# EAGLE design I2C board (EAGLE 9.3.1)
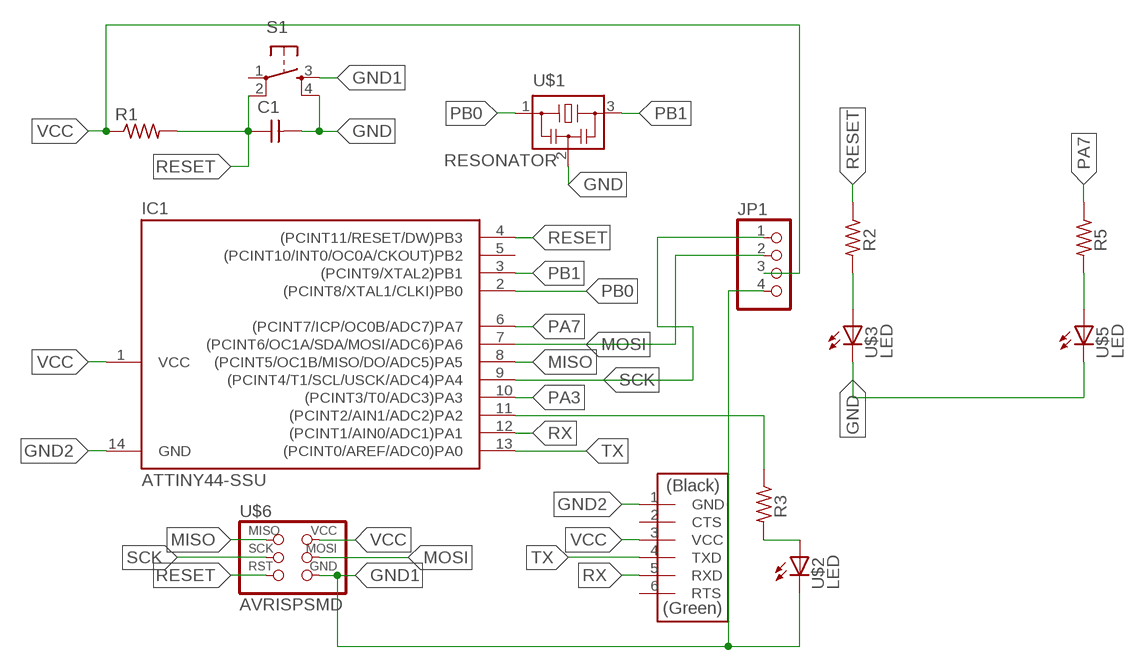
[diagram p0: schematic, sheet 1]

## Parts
C1  CAP-UNPOLARIZED  [C1206]
IC1  ATTINY44-SSU  [SOIC14]
JP1  PINHD-1X4  [1X04]
R1  RES-US1206  [R1206]
R2  RES-US1206  [R1206]
R3  RES-US1206  [R1206]
R5  RES-US1206  [R1206]
S1  6MM_SWITCH6MM_SWITCH  [6MM_SWITCH]
U$1  RESONATOR  [EFOBM]
U$2  LED  [LED1206]
U$3  LED  [LED1206]
U$5  LED  [LED1206]
U$6  AVRISPSMD  [2X03SMD]
U$7  FTDI-SMD-HEADER  [1X06SMD]

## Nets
GND: C1.2 S1.4(S1) U$1.2 U$3.2(C) U$5.2(C)
GND1: JP1.4 S1.3(S) U$2.2(C) U$6.6(GND)
GND2: IC1.14(GND) U$7.1(GND)
MISO: IC1.8((PCINT5/OC1B/MISO/DO/ADC5)PA5) U$6.1(MISO)
MOSI: IC1.7((PCINT6/OC1A/SDA/MOSI/ADC6)PA6) JP1.2 U$6.4(MOSI)
N$1: R3.2 U$2.1(A)
N$14: IC1.11((PCINT2/AIN1/ADC2)PA2) R3.1
N$20: R2.2 U$3.1(A)
N$23: R5.2 U$5.1(A)
PA3: IC1.10((PCINT3/T0/ADC3)PA3)
PA7: IC1.6((PCINT7/ICP/OC0B/ADC7)PA7) R5.1
PB0: IC1.2((PCINT8/XTAL1/CLKI)PB0) U$1.1
PB1: IC1.3((PCINT9/XTAL2)PB1) U$1.3
RESET: C1.1 IC1.4((PCINT11/RESET/DW)PB3) R1.2 R2.1 S1.2(P1) U$6.5(RST)
RX: IC1.12((PCINT1/AIN0/ADC1)PA1) U$7.5(RXD)
SCK: IC1.9((PCINT4/T1/SCL/USCK/ADC4)PA4) JP1.1 U$6.3(SCK)
TX: IC1.13((PCINT0/AREF/ADC0)PA0) U$7.4(TXD)
VCC: IC1.1(VCC) JP1.3 R1.1 U$6.2(VCC) U$7.3(VCC)
Unconnected: IC1.5((PCINT10/INT0/OC0A/CKOUT)PB2) S1.1(P) U$7.2(CTS) U$7.6(RTS)

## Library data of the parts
C1 = eagle_fab:CAP-UNPOLARIZED
IC1 = eagle_fab:ATTINY44
JP1 = pinhead:PINHD-1X4: PIN HEADER
R1-R3 R5 = eagle_fab:RES-US: Resistor (US Symbol)
S1 = eagle_fab:6MM_SWITCH: OMRON SWITCH
U$1 = eagle_fab:RESONATOR
U$2 U$3 U$5 = eagle_fab:LED: LED
U$6 = eagle_fab:AVRISP
U$7 = eagle_fab:FTDI-SMD-HEADER

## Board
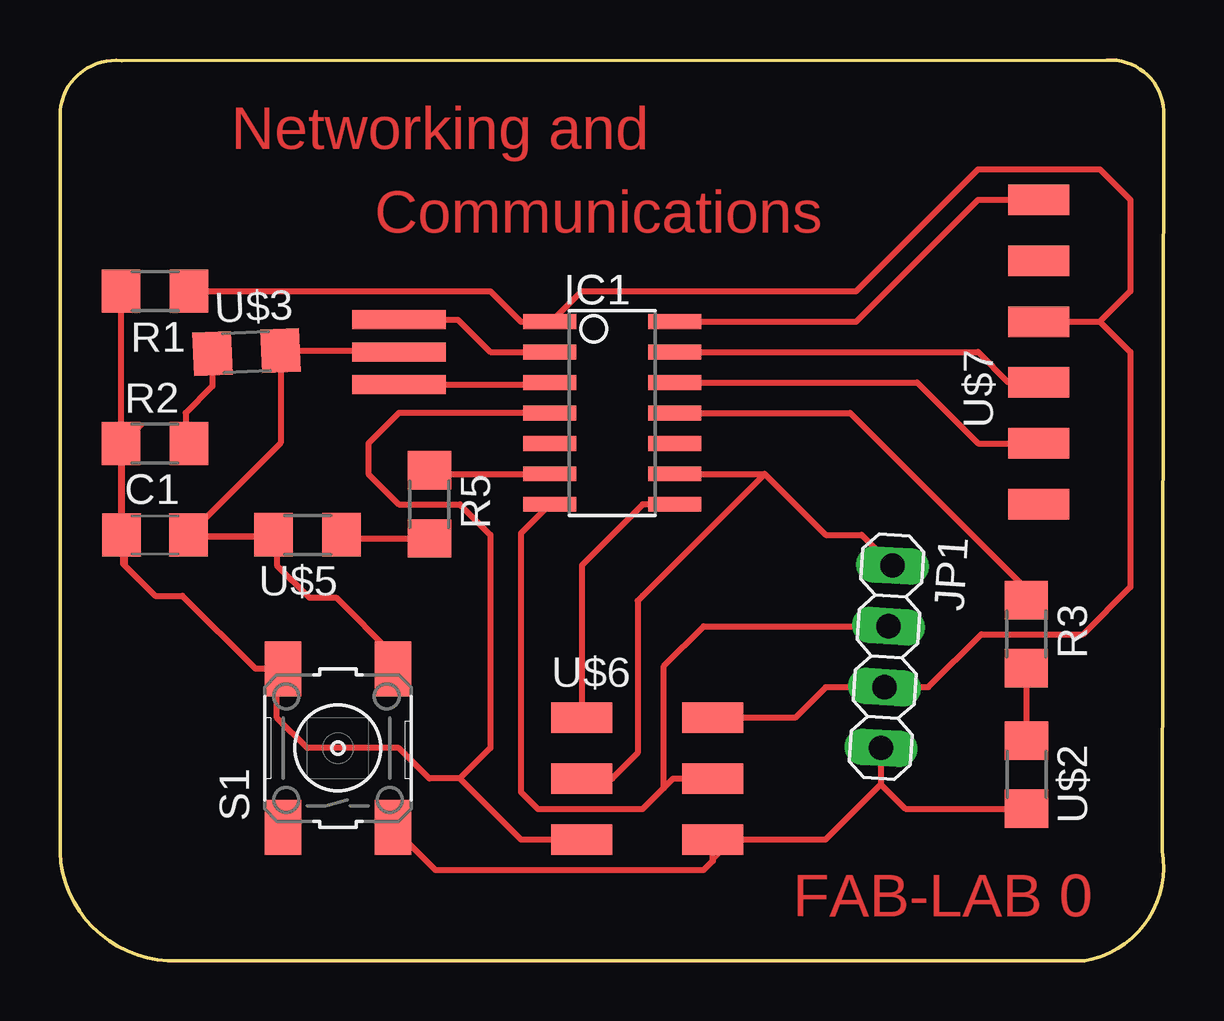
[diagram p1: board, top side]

Size 45.99 x 37.55 mm. Coordinates in mm from the lower left corner, seen from the top.
Outline: 0,35.44 arc-90 2.57,37.52 43.61,37.55 arc-90 45.99,35.44 45.93,4.59 arc-90 42.7,0 4.49,0.01 arc-90 0,4.96 0,35.44
Copper layers (1*16): Top 0.035mm / dielectric 1.5mm / Bottom 0.035mm
Design rules "default": minimum track width 6mil, minimum drill 0.35mm, track to track 6mil, track to pad 6mil, pad to pad 6mil, via to via 6mil, smd to smd 6mil, copper to edge 40mil, drill to drill 6mil, minimum pad ring 10mil, minimum via ring 8mil, stop-mask expansion 4mil, vias tented up to drill 0mil, thermal gap 10mil

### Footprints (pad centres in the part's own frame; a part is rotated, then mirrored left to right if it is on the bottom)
C1206 = smd 1.6 x 1.8: 1 -1.4,0; 2 1.4,0
SOIC14 = smd 0.61 x 2.21: 1 -3.81,-2.603; 2 -2.54,-2.603; 3 -1.27,-2.603; 4 0,-2.603; 5 1.27,-2.603; 6 2.54,-2.603; 7 3.81,-2.603; 8 3.81,2.603; 9 2.54,2.603; 10 1.27,2.603; 11 0,2.603; 12 -1.27,2.603; 13 -2.54,2.603; 14 -3.81,2.603
1X04 = drill 1.016 long: 1 -3.81,0; 2 -1.27,0; 3 1.27,0; 4 3.81,0
R1206 = smd 1.6 x 1.803: 1 -1.422,0; 2 1.422,0
6MM_SWITCH = smd 2.286 x 1.524: 1 -3.302,2.286; 2 3.302,2.286; 3 -3.302,-2.286; 4 3.302,-2.286
EFOBM = smd 0.8 x 3.9: 1 -1.35,0; 2 0,0; 3 1.35,0
LED1206 = smd 1.6 x 1.803: 1 -1.422,0; 2 1.422,0
2X03SMD = smd 2.54 x 1.27: 1 -2.54,2.54; 2 2.92,2.54; 3 -2.54,0; 4 2.92,0; 5 -2.54,-2.54; 6 2.92,-2.54
1X06SMD = smd 2.54 x 1.27: 1 0,6.35; 2 0,3.81; 3 0,1.27; 4 0,-1.27; 5 0,-3.81; 6 0,-6.35

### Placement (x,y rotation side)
C1  3.96,17.75 0 top
IC1  23.01,22.83 270 top
JP1  34.44,12.67 266.4 top
R1  3.96,27.91 180 top
R2  3.96,21.56 0 top
R3  40.26,13.62 270 top
R5  15.39,19.02 270 top
S1  11.58,8.86 90 top
U$1  14.12,25.37 270 top
U$2  40.27,7.76 270 top
U$3  7.77,25.37 2.5 top
U$5  10.31,17.75 180 top
U$6  24.28,7.59 0 top
U$7  40.79,25.37 0 top

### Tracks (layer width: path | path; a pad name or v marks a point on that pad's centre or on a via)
GND
  Top 0.152: U$3.2 8.89,25.13 | C1.2 U$5.2 8.96,17.68
  Top 0.254: U$1.2 14.06,25.44 U$3.2 9.19,21.59 C1.2 5.44,17.68 8.96,17.68 | U$5.2 9.04,17.6 9.04,16.48 10.39,15.14 11.5,15.14 13.87,12.78 S1.4
GND1
  Top 0.152: 26.82,3.78 28.09,5.05 | 28.09,5.05 31.9,5.05 | U$6.6 28.09,5.05
  Top 0.254: S1.3 15.64,3.78 26.82,3.78 27.2,4.16 U$6.6 31.9,5.05 34.2,7.36 | JP1.4 34.2,7.36 | 34.2,7.36 35.22,6.34 U$2.2
GND2
  Top 0.152: 25.55,26.64 IC1.14
  Top 0.254: IC1.14 33.17,26.64 38.25,31.72 U$7.1
MISO
  Top 0.254: IC1.8 24.28,19.02 21.74,16.48 U$6.1
MOSI
  Top 0.152: 34.44,13.94 JP1.2
  Top 0.254: IC1.7 19.2,17.82 19.2,7.04 19.91,6.32 24.28,6.32 25.16,7.2 | 34.44,13.94 26.82,13.94 25.16,12.28 25.16,7.2 | 25.16,7.2 25.55,7.59 U$6.4
N$1
  Top 0.254: R3.2 40.26,9.05 40.27,9.04 | 40.57,8.75 40.27,9.04 | 40.27,9.04 U$2.1
N$14
  Top 0.254: IC1.11 32.92,22.83 40.26,15.49 R3.1
N$20
  Top 0.152: 5.31,21.64 R2.2
  Top 0.254: U$3.1 6.35,23.95 5.23,22.83 5.23,21.72 5.31,21.64
N$23
  Top 0.254: U$5.1 11.88,17.6 R5.2
PA7
  Top 0.254: R5.1 15.54,20.29 IC1.6
PB0
  Top 0.254: U$1.1 16.58,26.72 17.93,25.37 IC1.2
PB1
  Top 0.152: U$1.3 14.2,24.1 | 20.33,24.02 IC1.3
  Top 0.254: U$1.3 20.33,24.02
RESET
  Top 0.152: S1.2 9.04,12.17 | 9.04,12.17 8.15,12.17 | C1.1 2.63,17.69 2.63,17.75 2.63,21.48 2.61,21.49 | R2.1 2.61,21.49 | 3.44,22.31 2.61,21.49 | 9.04,10.13 9.04,12.17
  Top 0.254: R1.2 R2.1 2.54,17.78 C1.1 2.69,17.62 2.69,16.48 | IC1.4 14.12,22.83 12.85,21.56 12.85,20.29 14.12,19.02 16.66,19.02 17.93,17.75 17.93,8.86 16.66,7.59 | 16.66,7.59 15.39,7.59 14.12,8.86 10.31,8.86 9.04,10.13 9.04,11.91 S1.2 8.15,12.17 5.1,15.21 3.96,15.21 2.69,16.48 | 2.63,17.75 2.63,16.55 2.69,16.48 | 16.66,7.59 19.2,5.05 U$6.5
RX
  Top 0.254: IC1.12 35.71,24.1 38.25,21.56 U$7.5
SCK
  Top 0.152: 34.56,16.6 JP1.1
  Top 0.254: IC1.9 29.36,20.29 | 29.36,20.29 31.9,17.75 33.4,17.75 34.56,16.6 | 29.36,20.29 24.28,15.21 24.07,15.01 24.07,8.66 23.01,7.59 U$6.3
TX
  Top 0.254: IC1.13 38.25,25.37 39.52,24.1 U$7.4
VCC
  Top 0.254: 43.33,26.64 44.6,27.91 44.6,31.72 43.33,32.99 38.25,32.99 33.17,27.91 21.74,27.91 20.47,26.64 IC1.1 19.2,26.64 17.93,27.91 R1.1 | JP1.3 | JP1.3 31.9,11.4 30.63,10.13 U$6.2 | JP1.3 | U$7.3 43.33,26.64 | 43.33,26.64 44.6,25.37 44.6,15.58 42.63,13.61 38.39,13.61 36.19,11.41 JP1.3 | 34.44,11.4 JP1.3
  Top 0.305: JP1.3 34.44,11.41 34.44,11.4

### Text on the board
Top: Networking and | Communications | FAB-LAB 0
